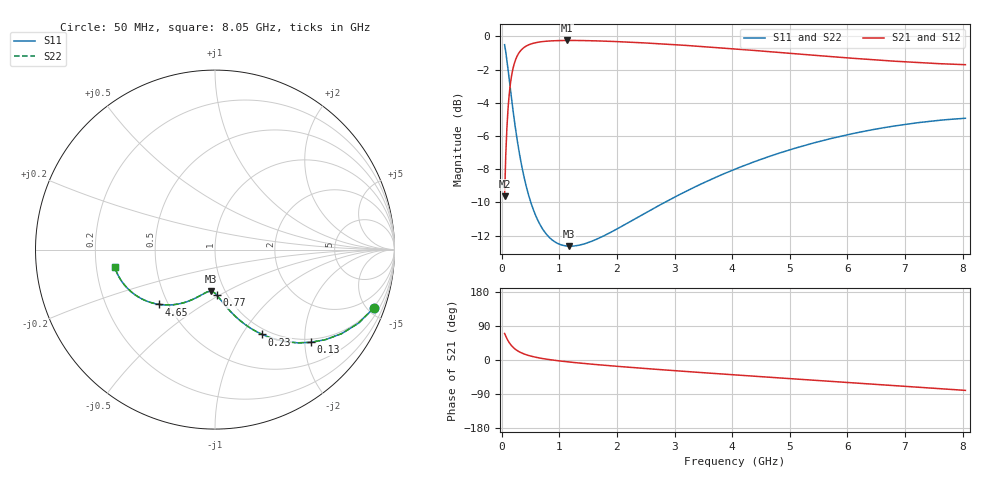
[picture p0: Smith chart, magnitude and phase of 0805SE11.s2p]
! AVX Thin Film Operation		Date: August 2001
! Description: Accu-P® Series, Thin Film, SMD, RF Capacitor
! Part Number: 08055J110FBT
! 50 MHz  -  8.05 GHz
! Serial Measurements
# mhz S db R 50
!	S11		S21		S12		S22
!	dB	Phase	dB	Phase	dB	Phase	dB	Phase
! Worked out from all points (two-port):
!   401 points, 50 MHz to 8.05 GHz, reference 50 ohm
!   highest |S21| = -0.25 dB at 1.13 GHz (marker M1); lowest = -9.6 dB at 50 MHz (marker M2)
!   |S21| within 3 dB of the highest: 137.8 MHz to end of sweep
!   lowest |S11| = -12.6 dB at 1.17 GHz (marker M3), VSWR 1.61, Z = 43.1 - j21.2 ohm
!   |S11| at or under -10 dB: 505.5 MHz to 2.827 GHz (2.322 GHz wide, 139 % of centre)
!   |S22| runs from -12.6 to -0.5 dB; largest |S21 - S12| = 0
!   S11 on the Smith chart (normalised r, x): 50 MHz: 0.92, -5.49; 130 MHz: 0.92, -2.13; 230 MHz: 0.92, -1.23; 770 MHz: 0.90, -0.49; 4.65 GHz: 0.45, -0.34; 8.05 GHz: 0.28, -0.08
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50  -0.50 -20.1  -9.62 69.9  -9.62 69.9  -0.50 -20.1
90  -1.44 -33.5  -5.50 56.5  -5.50 56.5  -1.44 -33.5
110  -2.00 -39.2  -4.33 50.8  -4.33 50.8  -2.00 -39.2
130  -2.58 -44.1  -3.49 45.9  -3.49 45.9  -2.58 -44.1
170  -3.74 -52.1  -2.39 37.8  -2.39 37.8  -3.74 -52.2
230  -5.34 -60.9  -1.51 29.1  -1.51 29.1  -5.34 -60.9
270  -6.28 -65.3  -1.17 24.7  -1.17 24.7  -6.28 -65.3
310  -7.11 -68.8  -0.94 21.2  -0.94 21.2  -7.11 -68.8
410  -8.81 -75.3  -0.61 14.7  -0.61 14.7  -8.81 -75.3
570  -10.63 -82.0  -0.40 7.9  -0.40 7.9  -10.63 -82.0
770  -11.89 -87.6  -0.29 2.4  -0.29 2.4  -11.89 -87.6
930  -12.39 -91.0  -0.26 -1.0  -0.26 -1.0  -12.39 -91.0
1130  -12.62 -94.5  -0.25 -4.6  -0.25 -4.6  -12.62 -94.5
1170  -12.63 -95.2  -0.25 -5.3  -0.25 -5.3  -12.63 -95.2
1390  -12.54 -98.5  -0.25 -8.6  -0.25 -8.6  -12.54 -98.5
2010  -11.58 -106.6  -0.32 -16.7  -0.32 -16.7  -11.58 -106.7
2730  -10.18 -115.0  -0.44 -25.1  -0.44 -25.1  -10.18 -115.0
4050  -8.00 -129.2  -0.76 -39.3  -0.76 -39.3  -8.00 -129.2
4650  -7.22 -135.4  -0.92 -45.5  -0.92 -45.5  -7.22 -135.4
5390  -6.44 -142.9  -1.13 -53.1  -1.13 -53.1  -6.44 -142.9
6730  -5.45 -156.4  -1.48 -66.6  -1.48 -66.6  -5.44 -156.4
8050  -4.93 -170.0  -1.71 -80.2  -1.71 -80.2  -4.93 -170.0
